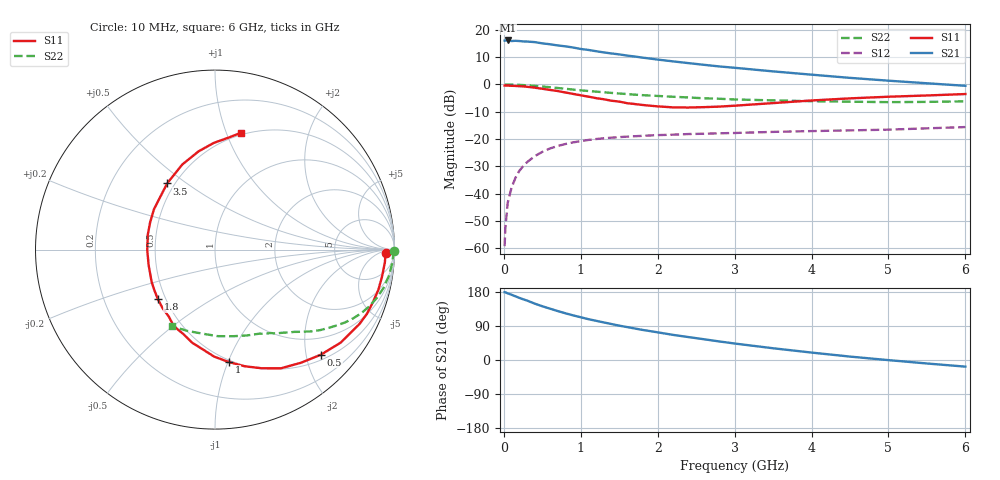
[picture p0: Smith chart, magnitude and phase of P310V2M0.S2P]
! SIEMENS Small Signal Semiconductors
! BFP181
! Si NPN RF Bipolar Junction Transistor in SOT143
! VCE = 10 V  IC = 2 mA
! Common Emitter S-Parameters:  March  1996
# GHz  S  MA  R  50
!  f  S11  S21  S12  S22
! GHz  MAG  ANG  MAG  ANG  MAG  ANG  MAG  ANG
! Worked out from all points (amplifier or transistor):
!   36 points, 10 MHz to 6 GHz, reference 50 ohm
!   highest |S21| = 16.1 dB at 50 MHz (marker M1)
!   |S21| within 3 dB of that: start of sweep to 978.4 MHz
!   unconditionally stable (mu >= 1): 2.605 GHz to end of sweep
!   at 250 MHz: K = 0.12, MSG = 22.8 dB, |S12| = -30.0 dB
!   at 1.4 GHz: K = 0.62, MSG = 15.4 dB, |S12| = -19.5 dB
!   at 6 GHz: K = 1.15, MAG = 5.2 dB, |S12| = -15.6 dB
!   S11 on the Smith chart (normalised r, x): 10 MHz: 35, -13; 500 MHz: 0.61, -2.30; 1 GHz: 0.48, -1.01; 1.8 GHz: 0.45, -0.30; 3.5 GHz: 0.46, +0.42; 6 GHz: 0.48, +1.13
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0.01  0.9507 -1.1  6.311 178.9  0.0011 80.0  0.9957 -0.4
0.02  0.9501 -1.9  6.341 178.6  0.0024 82.0  0.9929 -0.9
0.05  0.9491 -4.3  6.359 175.9  0.0068 85.8  0.9929 -2.2
0.1  0.9427 -9.2  6.205 172.2  0.0129 83.3  0.99 -4.4
0.15  0.9372 -13.9  6.267 168.1  0.0194 80.2  0.9845 -6.5
0.3  0.9052 -27.3  6.079 157.0  0.0376 72.5  0.9624 -12.9
0.4  0.8711 -36.5  5.931 148.9  0.0486 68.0  0.9398 -16.8
0.5  0.8316 -44.7  5.63 141.8  0.0583 62.5  0.9139 -20.4
0.6  0.7921 -52.7  5.418 135.5  0.0673 58.2  0.8881 -23.6
0.8  0.7106 -68.5  4.964 123.3  0.0812 50.5  0.8319 -29.1
0.9  0.6704 -75.8  4.726 117.8  0.087 47.0  0.8029 -31.6
1  0.6311 -83.0  4.442 112.8  0.0916 44.1  0.7786 -33.7
1.1  0.5964 -90.4  4.264 107.7  0.0964 41.4  0.7571 -35.6
1.3  0.5345 -103.7  3.842 99.1  0.1035 36.5  0.7169 -39.2
1.5  0.4844 -118.3  3.537 90.6  0.1085 33.0  0.6809 -42.1
1.8  0.421 -139.2  3.091 79.5  0.1145 29.0  0.6361 -46.1
2.2  0.3797 -166.8  2.635 66.3  0.1204 24.4  0.5935 -51.4
2.8  0.3922 157.1  2.13 49.0  0.1276 19.5  0.5462 -59.3
3.5  0.4549 125.9  1.729 31.0  0.1353 15.7  0.5102 -69.7
4.5  0.555 99.5  1.316 9.0  0.1442 11.0  0.4824 -88.3
5.5  0.6268 83.4  1.048 -9.2  0.1571 9.2  0.4785 -108.7
6  0.6661 77.5  0.942 -17.5  0.1658 7.2  0.49 -119.4
